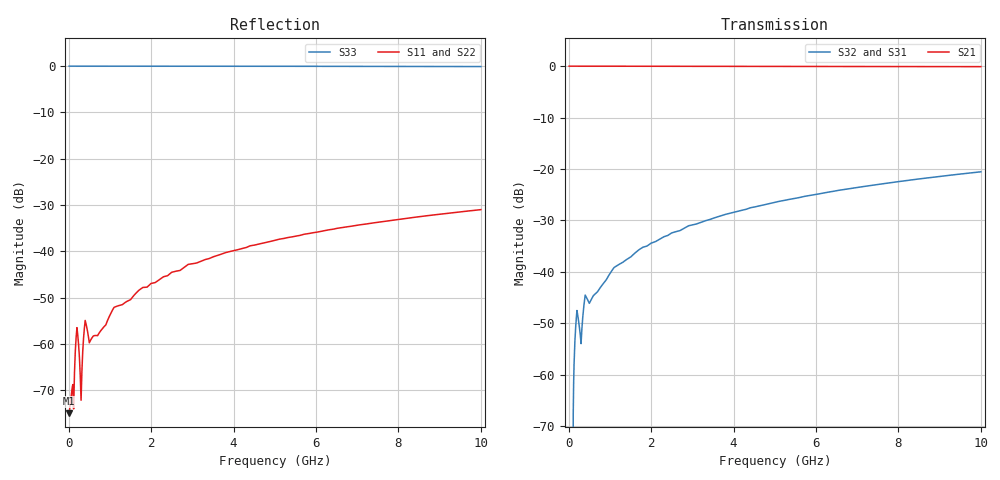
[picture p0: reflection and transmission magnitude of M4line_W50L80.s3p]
! Created Fri Sep 09 13:37:54 2011
# ghz S ma R 50
! 3 Port Network Data from SP1.SP block
! freq  magS11  angS11  magS12  angS12  magS13  angS13
!  magS21  angS21
!  magS22  angS22  magS23  angS23
!  magS31  angS31  magS32  angS32
!  magS33  angS33
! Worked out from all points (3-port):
!   1000 points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, 10 MHz to 10 GHz, reference 50 ohm
!   strongest paths, dB at 10 MHz, 2.51 GHz, 5.01 GHz, 7.51 GHz, 10 GHz:
!     S21: 0.0, 0.0, 0.0, -0.1, -0.1
!     S32: -, -32.4, -26.5, -23.0, -20.5
!     S31: -, -32.4, -26.5, -23.0, -20.5
!   lowest |S11| = -75.0 dB at 10 MHz (marker M1), VSWR 1.00, Z = 50 + j0.00322 ohm
!   |S11| at or under -10 dB: start of sweep to end of sweep
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0.01  0.0001782 10.4  0.9998 -0.0  0 0.0
      0.9998 -0.0  0.0001782 10.4  0 0.0
      0 0.0  0 0.0  1 0.0
0.07  0.0002983 35.2  0.9998 -0.0  0 0.0
      0.9998 -0.0  0.0002983 35.2  0 0.0
      0 0.0  0 0.0  1 0.0
0.18  0.001176 -80.3  0.9998 -0.1  0.00336 89.7
      0.9998 -0.1  0.001176 -80.3  0.00336 89.7
      0.00336 89.7  0.00336 89.7  1 -0.4
0.22  0.001242 -80.9  0.9998 -0.1  0.00376 89.7
      0.9998 -0.1  0.001242 -80.9  0.00376 89.7
      0.00376 89.7  0.00376 89.7  1 -0.4
0.3  0.0002464 -24.3  0.9998 -0.1  0.002 89.8
     0.9998 -0.1  0.0002464 -24.3  0.002 89.8
     0.002 89.8  0.002 89.8  1 -0.2
0.42  0.001648 -81.5  0.9997 -0.2  0.005733 89.5
      0.9997 -0.2  0.001648 -81.5  0.005733 89.5
      0.005733 89.5  0.005733 89.5  1 -0.7
0.54  0.001117 -74.5  0.9997 -0.2  0.005306 89.5
      0.9997 -0.2  0.001117 -74.5  0.005306 89.5
      0.005306 89.5  0.005306 89.5  1 -0.6
1.79  0.004051 -76.2  0.9987 -0.8  0.01723 88.5
      0.9987 -0.8  0.004051 -76.2  0.01723 88.5
      0.01723 88.5  0.01723 88.5  0.9997 -2.0
5.01  0.01317 -83.0  0.9955 -2.0  0.04739 85.8
      0.9955 -2.0  0.01317 -83.0  0.04739 85.8
      0.04739 85.8  0.04739 85.8  0.9975 -5.4
10  0.02822 -91.2  0.9891 -3.7  0.09387 81.7
    0.9891 -3.7  0.02822 -91.2  0.09387 81.7
    0.09387 81.7  0.09387 81.7  0.9905 -10.8
